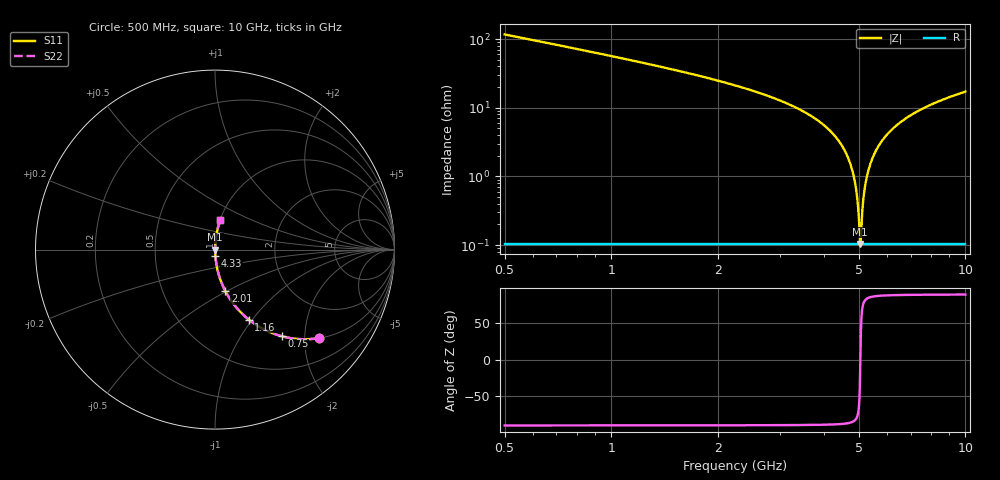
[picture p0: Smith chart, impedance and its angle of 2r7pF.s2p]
! Created Fri Jan 10 15:51:52 2014
# hz S db R 50
! 2 Port Network Data from SP1.SP block
! freq  dbS11  angS11  dbS21  angS21  dbS12  angS12  dbS22  angS22
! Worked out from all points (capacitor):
!   951 points, 500 MHz to 10 GHz, reference 50 ohm
!   read as one part in series: C = 2.7 pF near 540 MHz
!   lowest |Z| = 104 mohm at 5.05 GHz (marker M1)
!   series resonance near 5.051 GHz, so ESL is about 370 pH
!   S11 on the Smith chart (normalised r, x): 500 MHz: 1.00, -2.33; 750 MHz: 1.00, -1.54; 1.16 GHz: 1.00, -0.96; 2.01 GHz: 1.00, -0.49; 4.33 GHz: 1.00, -0.07; 10 GHz: 1.00, +0.34
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5e8  -2.39 -40.6  -3.74 49.4  -3.74 49.4  -2.39 -40.6
7.5e8  -4.31 -52.4  -2.02 37.5  -2.02 37.5  -4.31 -52.4
1.16e9  -7.26 -64.2  -0.91 25.7  -0.91 25.7  -7.26 -64.2
2.01e9  -12.42 -75.9  -0.27 13.9  -0.27 13.9  -12.42 -75.9
2.09e9  -12.86 -76.6  -0.24 13.1  -0.24 13.1  -12.86 -76.6
3.67e9  -22.44 -84.9  -0.03 4.3  -0.03 4.3  -22.44 -84.9
4.33e9  -28.86 -86.3  -0.01 2.1  -0.01 2.1  -28.86 -86.3
4.62e9  -33.62 -86.0  -0.01 1.2  -0.01 1.2  -33.62 -86.0
4.82e9  -39.19 -83.9  -0.01 0.6  -0.01 0.6  -39.19 -83.9
4.93e9  -44.80 -79.3  -0.01 0.3  -0.01 0.3  -44.80 -79.3
4.97e9  -48.14 -74.4  -0.01 0.2  -0.01 0.2  -48.14 -74.4
5.02e9  -55.00 -54.2  -0.01 0.1  -0.01 0.1  -55.00 -54.2
5.05e9  -59.66 -3.0  -0.01 0.0  -0.01 0.0  -59.66 -3.0
5.08e9  -55.47 51.9  -0.01 -0.1  -0.01 -0.1  -55.47 51.9
5.16e9  -45.89 77.9  -0.01 -0.3  -0.01 -0.3  -45.89 77.9
5.25e9  -40.85 82.9  -0.01 -0.5  -0.01 -0.5  -40.85 82.9
5.46e9  -34.80 85.7  -0.01 -1.0  -0.01 -1.0  -34.80 85.7
5.77e9  -30.14 86.3  -0.01 -1.8  -0.01 -1.8  -30.14 86.3
6.22e9  -26.23 86.0  -0.02 -2.8  -0.02 -2.8  -26.23 86.0
6.84e9  -22.90 85.1  -0.03 -4.1  -0.03 -4.1  -22.90 85.1
8.42e9  -18.17 82.4  -0.08 -7.1  -0.08 -7.1  -18.17 82.4
1e10  -15.42 79.9  -0.14 -9.8  -0.14 -9.8  -15.42 79.9
